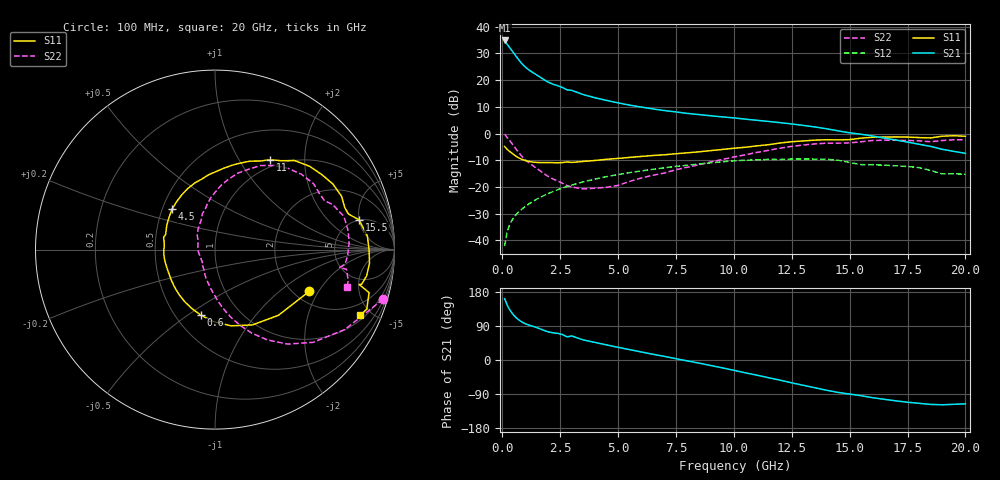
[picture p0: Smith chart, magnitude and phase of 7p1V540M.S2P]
! Infineon Technologies  Discrete & RF Semiconductors
! bfp620
! VCE =  1.5 V,  IC =  40 mA
! Common Emitter S-Parameters:  Sep 2002
# GHz  S  MA  R  50
!  f  S11  S21  S12  S22
! GHz  MAG  ANG  MAG  ANG  MAG  ANG  MAG  ANG
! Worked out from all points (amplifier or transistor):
!   59 points, 100 MHz to 20 GHz, reference 50 ohm
!   highest |S21| = 34.8 dB at 100 MHz (marker M1)
!   |S21| within 3 dB of that: start of sweep to 347.1 MHz
!   unconditionally stable (mu >= 1): 2.752 GHz to 2.902 GHz; 3.095 GHz to 9.851 GHz; 17.18 GHz to end of sweep
!   at 1 GHz: K = 0.82, MSG = 26.0 dB, |S12| = -27.3 dB
!   at 5.5 GHz: K = 1.04, MAG = 11.5 dB, |S12| = -14.6 dB
!   at 20 GHz: K = 1.31, MAG = 0.6 dB, |S12| = -15.3 dB
!   S11 on the Smith chart (normalised r, x): 100 MHz: 2.39, -1.66; 600 MHz: 0.66, -0.57; 4.5 GHz: 0.56, +0.29; 11 GHz: 0.90, +1.37; 15.5 GHz: 4.93, +4.98; 20 GHz: 1.23, -4.29
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0.1  0.5736 -24.0  55.12 161.9  0.0078 82.4  0.9758 -16.5
0.2  0.5089 -46.0  47.35 146.7  0.0139 72.5  0.8497 -31.6
0.3  0.4686 -63.6  41.51 134.7  0.0189 68.3  0.7519 -43.4
0.4  0.4339 -78.1  36.4 125.4  0.0232 65.8  0.6635 -52.5
0.5  0.402 -90.7  31.78 117.8  0.027 64.1  0.5818 -59.9
0.6  0.3744 -101.9  27.7 111.6  0.0305 63.0  0.5087 -66.2
0.7  0.3521 -111.8  24.24 106.4  0.0338 62.2  0.4461 -71.5
0.9  0.3219 -127.9  19.18 98.5  0.0402 61.3  0.353 -79.9
1.1  0.304 -139.4  16.06 93.2  0.0465 60.7  0.294 -85.9
1.3  0.2931 -148.3  14.02 89.2  0.053 60.1  0.2537 -90.7
2  0.2863 -174.3  9.072 74.0  0.0758 56.2  0.1557 -110.5
2.8  0.2943 166.7  6.553 61.1  0.1021 50.1  0.1059 -134.5
3  0.2876 162.9  6.417 63.4  0.1085 48.4  0.0997 -134.3
3.5  0.3007 153.4  5.342 52.9  0.1248 43.9  0.0919 -153.4
4.5  0.329 136.6  4.166 39.9  0.1559 34.5  0.0984 165.3
7  0.4001 100.5  2.691 9.6  0.2282 10.0  0.1824 114.8
10.5  0.5537 63.0  1.857 -33.9  0.3162 -29.7  0.4006 78.9
11  0.5871 58.5  1.766 -40.1  0.3216 -35.3  0.4438 73.5
13.5  0.7517 29.1  1.327 -73.2  0.332 -66.0  0.6387 41.1
15.5  0.8193 11.7  0.969 -94.2  0.2616 -88.2  0.7018 20.9
17  0.8642 -5.1  0.757 -107.8  0.2488 -97.7  0.7479 2.6
20  0.8887 -24.4  0.425 -115.7  0.1726 -107.7  0.7642 -15.9
